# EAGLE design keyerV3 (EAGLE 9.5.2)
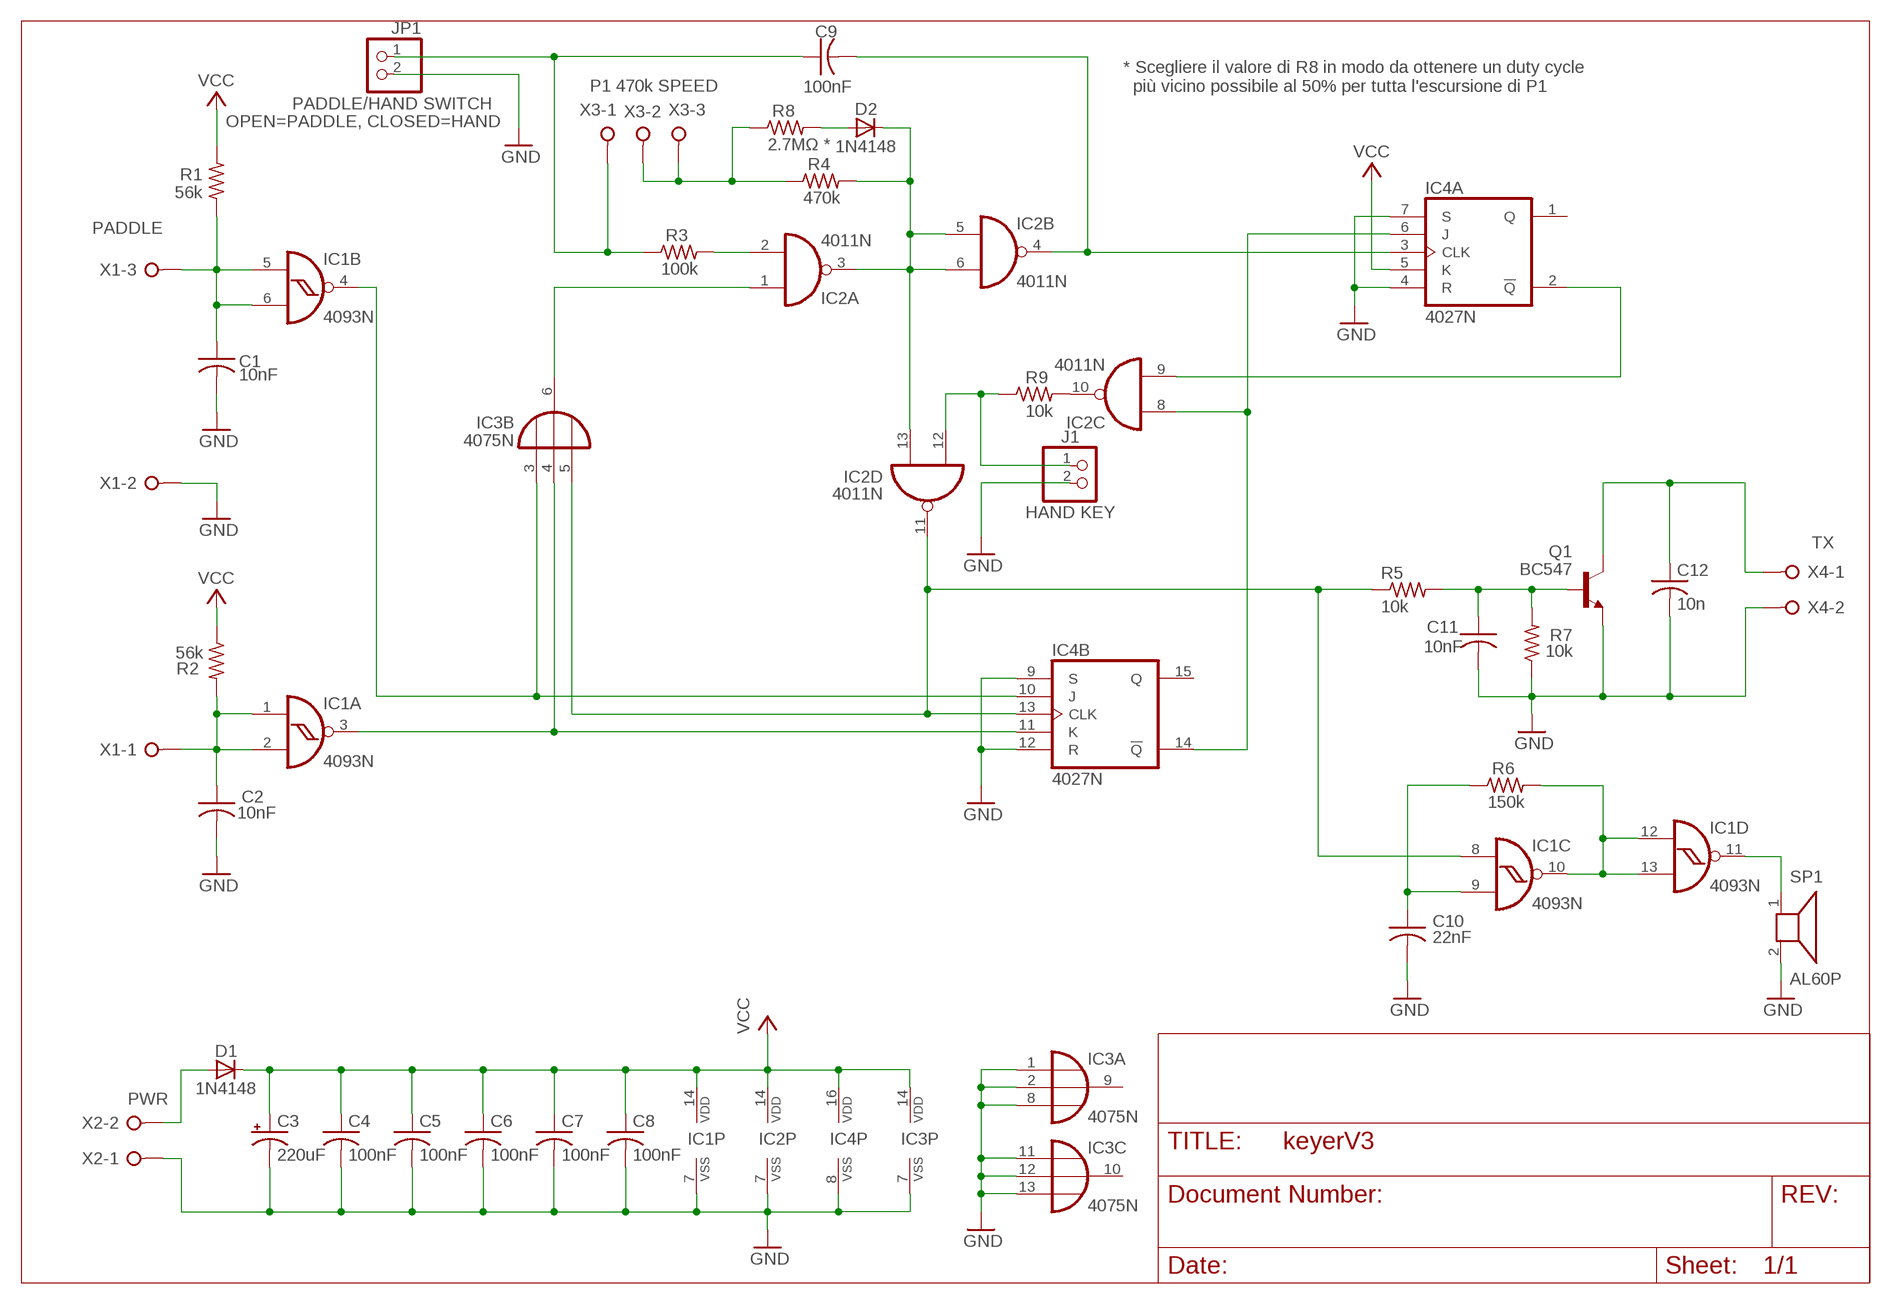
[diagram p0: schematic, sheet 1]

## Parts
C1  10nF  C-US050-025X075  [C050-025X075]
C2  10nF  C-US050-025X075  [C050-025X075]
C3  220uF  CPOL-USE5-8.5  [E5-8,5]
C4  100nF  C-US050-025X075  [C050-025X075]
C5  100nF  C-US050-025X075  [C050-025X075]
C6  100nF  C-US050-025X075  [C050-025X075]
C7  100nF  C-US050-025X075  [C050-025X075]
C8  100nF  C-US050-025X075  [C050-025X075]
C9  100nF  C-US102-043X133  [C102-043X133]
C10  22nF  C-US050-025X075  [C050-025X075]
C11  10nF  C-US050-025X075  [C050-025X075]
C12  10n  C-US050-025X075  [C050-025X075]
D1  1N4148  1N4148DO35-7  [DO35-7]
D2  1N4148  1N4148DO35-7  [DO35-7]
IC1  4093N  [DIL14]
IC2  4011N  [DIL14]
IC3  4075N  [DIL14]
IC4  4027N  [DIL16]
J1  HAND KEY  PINHD-1X2  [1X02]
JP1  PADDLE/HAND SWITCH  PINHD-1X2  [1X02]
Q1  BC547  [TO92]
R1  56k  R-US_0207/10  [0207/10]
R2  56k  R-US_0207/10  [0207/10]
R3  100k  R-US_0207/10  [0207/10]
R4  470k  R-US_0207/10  [0207/10]
R5  10k  R-US_0207/10  [0207/10]
R6  150k  R-US_0207/10  [0207/10]
R7  10k  R-US_0207/10  [0207/10]
R8  2.7MΩ *  R-US_0207/10  [0207/10]
R9  10k  R-US_0207/10  [0207/10]
SP1  AL60P  [AL60P]
X1  PADDLE  W237-03P  [W237-133]
X2  PWR  W237-02P  [W237-132]
X3  P1 470k SPEED  W237-03P  [W237-133]
X4  TX  W237-02P  [W237-132]

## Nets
GND: C1.2 C2.2 C3.- C4.2 C5.2 C6.2 C7.2 C8.2 C10.2 C11.2 C12.2 IC1.7(P:VSS) IC2.7(P:VSS) IC3.1(A:I0) IC3.2(A:I1) IC3.7(P:VSS) IC3.8(A:I2) IC3.11(C:I0) IC3.12(C:I1) IC3.13(C:I2) IC4.4(A:R) IC4.7(A:S) IC4.8(P:VSS) IC4.9(B:S) IC4.12(B:R) J1.2 JP1.2 Q1.1(E) R7.1 SP1.2 X1.2 X2.1 X4.2
N$1: C1.1 IC1.5(B:I0) IC1.6(B:I1) R1.1 X1.3
N$2: C2.1 IC1.1(A:I0) IC1.2(A:I1) R2.2 X1.1
N$3: IC1.4(B:O) IC3.3(B:I0) IC4.10(B:J)
N$4: IC2.1(A:I0) IC3.6(B:O)
N$5: IC2.2(A:I1) R3.2
N$6: C9.1 JP1.1 R3.1 X3.1
N$7: R4.1 R8.1 X3.2 X3.3
N$8: D2.C IC2.3(A:O) IC2.5(B:I0) IC2.6(B:I1) IC2.13(D:I1) R4.2
N$9: C9.2 IC2.4(B:O) IC4.3(A:CLK)
N$10: IC1.11(D:O) SP1.1
N$11: IC1.3(A:O) IC3.4(B:I1) IC4.11(B:K)
N$12: D1.A X2.2
N$13: IC2.10(C:O) R9.2
N$14: IC1.8(C:I0) IC2.11(D:O) IC3.5(B:I2) IC4.13(B:CLK) R5.1
N$15: D2.A R8.2
N$16: IC2.8(C:I0) IC4.6(A:J) IC4.14(B:!Q)
N$17: IC2.9(C:I1) IC4.2(A:!Q)
N$18: IC1.10(C:O) IC1.12(D:I0) IC1.13(D:I1) R6.2
N$19: C10.1 IC1.9(C:I1) R6.1
N$20: IC2.12(D:I0) J1.1 R9.1
N$21: C11.1 Q1.2(B) R5.2 R7.2
N$24: C12.1 Q1.3(C) X4.1
VCC: C3.+ C4.1 C5.1 C6.1 C7.1 C8.1 D1.C IC1.14(P:VDD) IC2.14(P:VDD) IC3.14(P:VDD) IC4.5(A:K) IC4.16(P:VDD) R1.2 R2.1
Unconnected: IC3.9(A:O) IC3.10(C:O) IC4.1(A:Q) IC4.15(B:Q)

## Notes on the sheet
- * Scegliere il valore di R8 in modo da ottenere un duty cycle
    più vicino possibile al 50% per tutta l'escursione di P1

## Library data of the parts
C1 C2 C4-C12 = rcl:C-US: CAPACITOR, American symbol
C3 = rcl:CPOL-US: POLARIZED CAPACITOR, American symbol
D1 D2 = diode:1N4148: DIODE
IC1 = 40xx:4093: Quad 2-input NAND schmitt trigger
IC2 = 40xx:4011: Quad 2-input NAND
IC3 = 40xx:4075: Triple 3-input OR
IC4 = 40xx:4027: Dual JK FLIP FLOP
J1 = pinhead:PINHD-1X2: PIN HEADER
JP1 = pinhead:PINHD-1X2: PIN HEADER; INFO: OPEN=PADDLE, CLOSED=HAND
Q1 = transistor-npn:BC547*: NPN Transistor
R1-R9 = rcl:R-US_: RESISTOR, American symbol
SP1 = buzzer:AL60P: SPEAKER; OC_FARNELL: unknown; OC_NEWARK: unknown
X1 X3 = con-wago-508:W237-03P: WAGO SREW CLAMP; OC_FARNELL: unknown; OC_NEWARK: unknown
X2 X4 = con-wago-508:W237-02P: WAGO SREW CLAMP; OC_FARNELL: unknown; OC_NEWARK: unknown

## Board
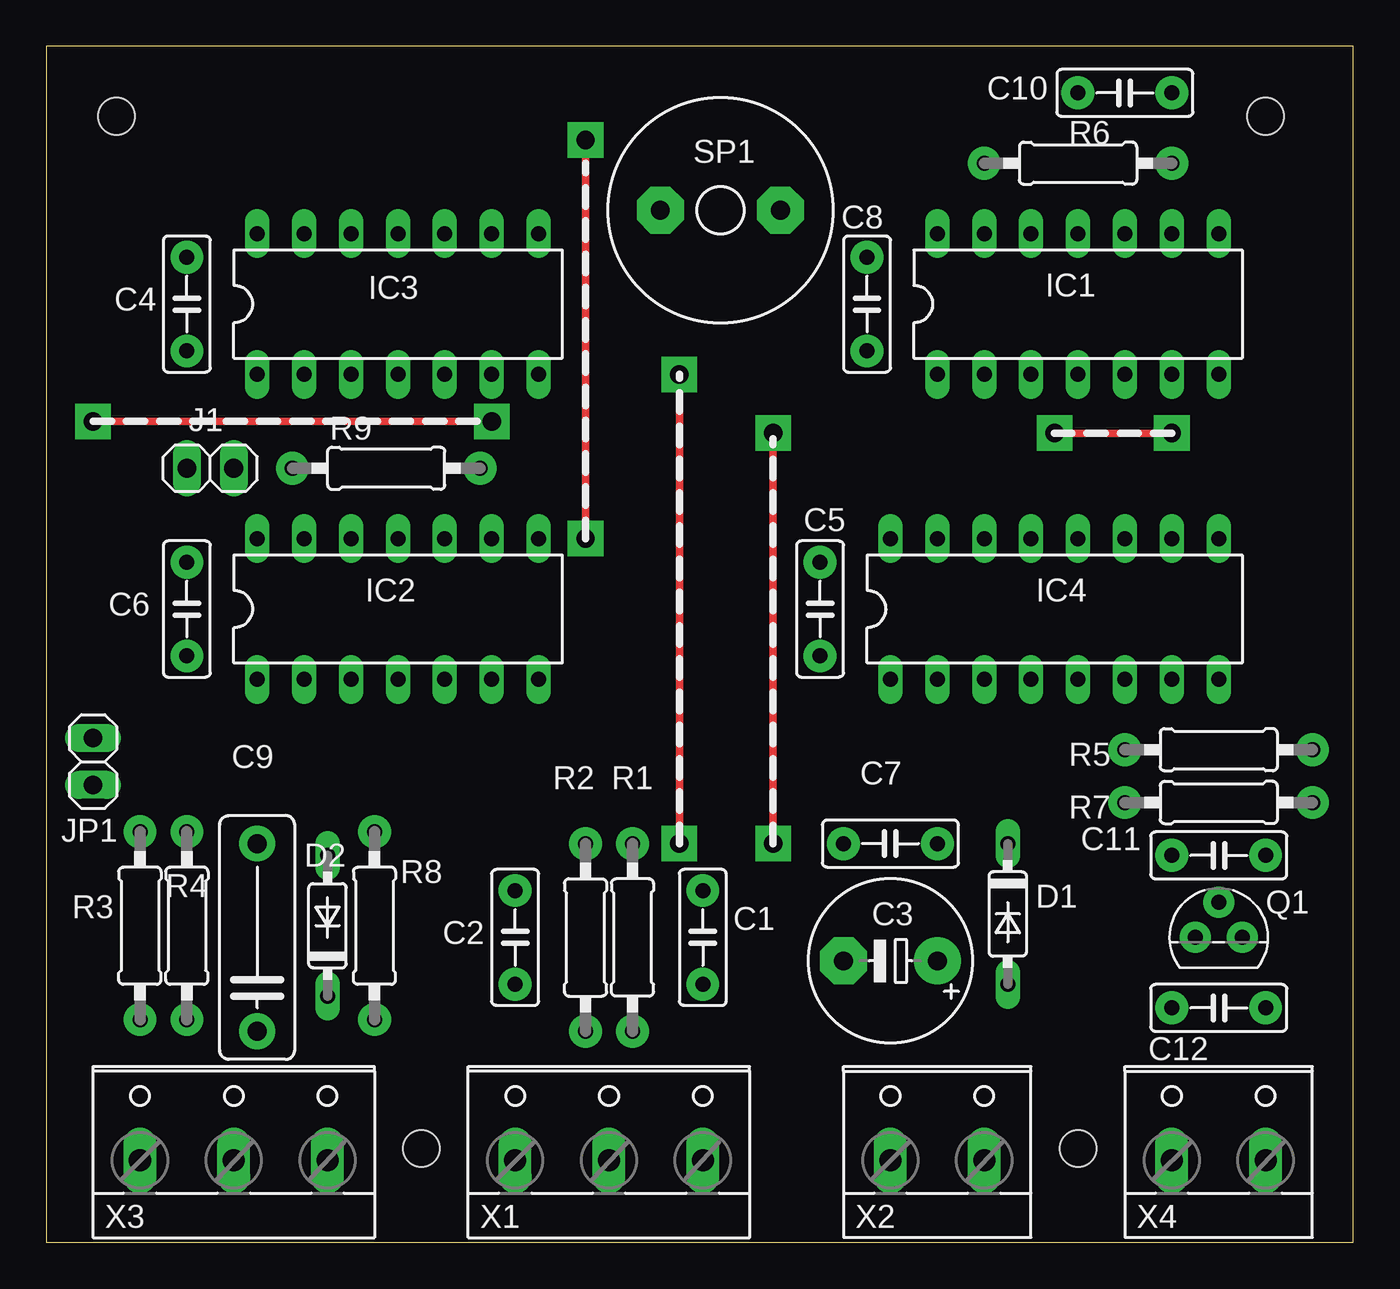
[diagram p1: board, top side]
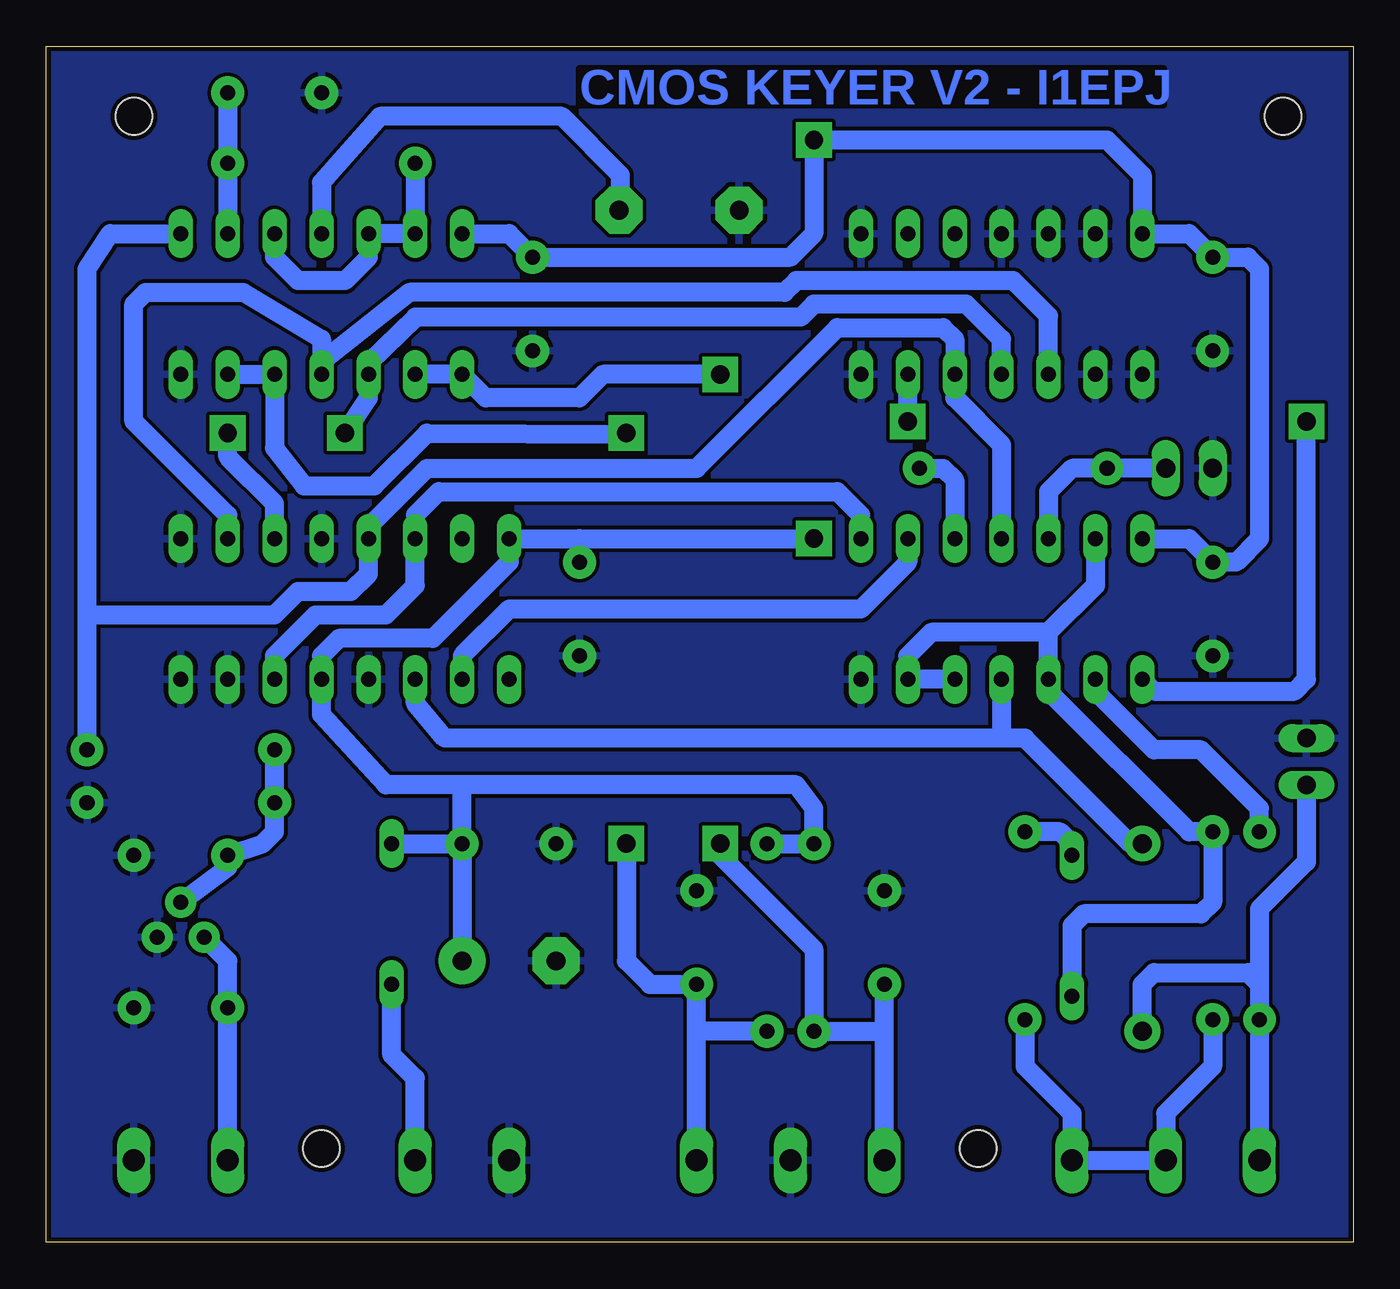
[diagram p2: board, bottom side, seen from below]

Size 70.79 x 64.76 mm. Coordinates in mm from the lower left corner, seen from the top.
Outline: 0,0 70.79,0 70.79,64.76 0,64.76 0,0
Copper layers (1*16): Top 0.035mm / dielectric 1.5mm / Bottom 0.035mm
Design rules "default *": minimum track width 10mil, minimum drill 24mil, track to track 8mil, track to pad 8mil, pad to pad 8mil, via to via 8mil, smd to smd 8mil, copper to edge 10mil, drill to drill 8mil, minimum pad ring 10mil, minimum via ring 8mil, stop-mask expansion 4mil, vias tented up to drill 0mil, thermal gap 10mil
Holes 2 mm at 3.81,60.96 66.04,60.96 20.32,5.08 55.88,5.08

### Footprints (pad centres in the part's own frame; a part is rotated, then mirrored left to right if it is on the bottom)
C050-025X075 = drill 0.813 pad 1.778: 1 -2.54,0; 2 2.54,0
E5-8,5 = drill 1.016 pad 2.54: + -2.54,0 | drill 1.016 pad 2.54 octagon: - 2.54,0
C102-043X133 = drill 1.016 pad 1.93: 1 -5.08,0; 2 5.08,0
DO35-7 = drill 0.813 long: A 3.81,0; C -3.81,0
DIL14 = drill 0.813 long: 1 -7.62,-3.81; 2 -5.08,-3.81; 3 -2.54,-3.81; 4 0,-3.81; 5 2.54,-3.81; 6 5.08,-3.81; 7 7.62,-3.81; 8 7.62,3.81; 9 5.08,3.81; 10 2.54,3.81; 11 0,3.81; 12 -2.54,3.81; 13 -5.08,3.81; 14 -7.62,3.81
DIL16 = drill 0.813 long: 1 -8.89,-3.81; 2 -6.35,-3.81; 3 -3.81,-3.81; 4 -1.27,-3.81; 5 1.27,-3.81; 6 3.81,-3.81; 7 6.35,-3.81; 8 8.89,-3.81; 9 8.89,3.81; 10 6.35,3.81; 11 3.81,3.81; 12 1.27,3.81; 13 -1.27,3.81; 14 -3.81,3.81; 15 -6.35,3.81; 16 -8.89,3.81
1X02 = drill 1.016 long: 1 -1.27,0; 2 1.27,0
TO92 = drill 0.813 pad 1.676: 1 1.27,0; 2 0,1.905; 3 -1.27,0
0207/10 = drill 0.813 pad 1.778: 1 -5.08,0; 2 5.08,0
AL60P = drill 1.016 pad 2.54 octagon: 1 -3.251,0; 2 3.251,0
W237-133 = drill 1.194 long: 1 -5.08,-0.635; 2 0,-0.635; 3 5.08,-0.635
W237-132 = drill 1.194 long: 1 -2.54,-0.635; 2 2.54,-0.635

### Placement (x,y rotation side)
C1  35.56,16.51 90 top
C2  25.4,16.51 90 top
C3  45.72,15.24 180 top
C4  7.62,50.8 270 top
C5  41.91,34.29 270 top
C6  7.62,34.29 270 top
C7  45.72,21.59 180 top
C8  44.45,50.8 270 top
C9  11.43,16.51 90 top
C10  58.42,62.23 180 top
C11  63.5,20.95 0 top
C12  63.5,12.7 0 top
D1  52.07,17.78 270 top
D2  15.24,17.14 90 top
IC1  55.88,50.8 0 top
IC2  19.05,34.29 0 top
IC3  19.05,50.8 0 top
IC4  54.61,34.29 0 top
J1  8.89,41.91 180 top
JP1  2.54,26.04 90 top
Q1  63.5,16.51 0 top
R1  31.75,16.51 90 top
R2  29.21,16.51 270 top
R3  5.08,17.14 90 top
R4  7.62,17.14 90 top
R5  63.5,26.67 180 top
R6  55.88,58.42 180 top
R7  63.5,23.81 180 top
R8  17.78,17.14 90 top
R9  18.41,41.91 0 top
SP1  36.51,55.88 180 top
X1  30.48,5.08 0 top
X2  48.26,5.08 0 top
X3  10.16,5.08 0 top
X4  63.5,5.08 0 top

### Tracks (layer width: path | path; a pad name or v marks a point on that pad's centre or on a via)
GND
  pour Bottom: 0,64.77 0,0 71.12,0 71.12,64.77
N$1  (via drill 1 pad 1.93)
  Top 0.406: v39.37,43.81 v39.37,21.59
  Bottom 1.016: R1.1 35.56,11.43 | X1.3 35.56,11.43 | 35.56,11.43 C1.1 38.1,13.97 39.37,15.24 v39.37,21.59 | IC1.6 IC1.5 58.42,43 56.83,40.96 53.02,40.96 50.17,43.81 39.44,43.75 v39.37,43.81
N$2  (via drill 1 pad 1.93)
  Top 0.406: v34.29,21.59 v34.29,46.99
  Bottom 1.016: X1.1 25.4,11.43 | 25.4,11.43 R2.2 29.21,15.88 34.29,20.95 v34.29,21.59 | 25.4,11.43 C2.1 | v34.29,46.99 40.64,46.99 41.91,45.72 46.99,45.72 IC1.1 IC1.2
N$3
  Bottom 1.016: 55.88,47.66 51.12,51.44 30.8,51.44 30.16,52.07 18.41,52.07 16.51,50.16 IC3.3 | IC4.10 60.96,39.37 66.04,44.45 66.04,50.8 65.41,51.44 60.11,51.44 55.88,48.9 55.88,47.66 | 55.88,47.66 IC1.4
N$4  (via drill 1 pad 1.93)
  Top 0.406: v24.13,44.45 v2.54,44.45
  Bottom 1.016: IC2.1 10.79,29.84 3.17,29.84 2.54,30.48 v2.54,44.45 | v24.13,44.45 IC3.6
N$5
  Bottom 1.016: R3.2 5.08,23.5 8.26,26.67 10.79,26.67 13.97,29.84 IC2.2
N$6
  Bottom 1.016: X3.1 R3.1 5.08,13.97 | C9.1 11.43,13.97 10.79,14.61 5.71,14.61 5.08,13.97 | 5.08,13.97 5.08,18.06 2.54,20.6 JP1.1
N$7
  Bottom 1.016: R8.1 17.78,9.53 15.24,6.99 X3.3 X3.2 10.16,6.99 7.62,9.53 R4.1
N$8
  Bottom 1.016: IC2.13 13.97,35.56 16.51,33.02 | 16.51,33.02 IC2.3 16.51,29.84 8.89,22.23 R4.2 7.62,18.41 8.26,17.78 14.61,17.78 15.24,17.14 D2.C | 16.51,33.02 22.86,33.02 24.13,31.75 IC2.6 IC2.5
N$9
  Bottom 1.016: IC2.4 19.05,27.3 | 19.05,27.3 17.78,27.3 12.06,21.59 C9.2 | 19.05,27.3 49.21,27.3 50.8,29.21 IC4.3
N$10
  Bottom 1.016: IC1.11 55.88,57.39 52.7,60.96 42.86,60.96 39.69,57.78 39.69,55.88 SP1.1
N$11  (via drill 1 pad 1.93)
  Top 0.406: v60.96,43.81 v54.61,43.81
  Bottom 1.016: IC3.4 19.05,48.9 20.95,50.8 29.21,50.8 29.92,50.09 50.79,50.09 53.34,47.62 IC1.3 53.34,45.72 v54.61,43.81 | IC4.11 58.42,40.01 60.96,42.55 v60.96,43.81
N$12
  Bottom 1.016: X2.2 50.8,8.89 52.07,10.16 D1.A
N$13
  Bottom 1.016: R9.2 22.23,41.91 21.59,41.27 IC2.10
N$14
  Bottom 1.016: IC2.11 19.05,43.18 21.59,45.72 IC3.5 21.59,48.9 22.23,49.53 27.94,49.53 35.56,41.91 50.16,41.91 53.34,38.73 IC4.13 53.34,36.2 54.29,35.24 57.15,35.24 58.42,33.97 68.58,33.97 | R5.1 68.58,33.97 | 68.58,33.97 68.58,52.7 67.31,54.61 IC1.8
N$15
  Bottom 1.016: D2.A 15.24,21.59 15.88,22.23 R8.2
N$16
  Bottom 0.406: IC4.14 50.8,39.37 | 26.67,39.37 IC2.8
  Bottom 1.016: 50.8,39.37 49.53,40.64 27.94,40.64 26.67,39.37 | IC4.6 58.42,31.75 56.2,33.97 52.39,33.97 50.8,35.56 IC4.14
N$17
  Bottom 1.016: IC2.9 24.13,36.83 26.67,34.29 45.72,34.29 48.26,31.75 IC4.2
N$18
  Bottom 0.406: IC1.12 53.34,53.34
  Bottom 1.016: R6.2 IC1.13 IC1.12 | 53.34,53.34 54.61,52.07 57.15,52.07 58.42,53.34 IC1.10
N$19
  Bottom 1.016: C10.1 R6.1 IC1.9
N$20
  Bottom 1.016: IC2.12 16.51,40.64 15.24,41.91 R9.1 J1.1
N$21
  Bottom 1.016: Q1.2 60.96,20.32 C11.1 59.05,21.59 58.42,22.23 R7.2 R5.2
N$24
  Bottom 1.016: X4.1 C12.1 60.96,15.24 Q1.3
VCC  (via drill 1 pad 1.93)
  Top 0.406: v29.21,38.1 v29.21,59.69
  Bottom 1.016: IC2.14 8.89,38.1 C6.1 6.35,36.83 5.08,38.1 5.08,52.7 5.71,53.34 C4.1 8.89,54.61 IC3.14 11.43,57.78 13.34,59.69 v29.21,59.69 29.21,54.61 30.48,53.34 C8.1 45.72,54.61 IC1.14 | C7.1 48.26,24.77 | 48.26,24.77 52.39,24.77 55.88,28.57 IC4.5 55.88,31.75 54.93,32.7 49.85,32.7 45.72,36.83 IC4.16 41.91,38.1 | C7.1 C3.+ | R1.2 R2.1 29.21,23.5 30.16,24.77 48.26,24.77 | 41.91,38.1 C5.1 | 41.91,38.1 v29.21,38.1 | D1.C C7.1

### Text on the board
Bottom: CMOS KEYER V2 - I1EPJ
